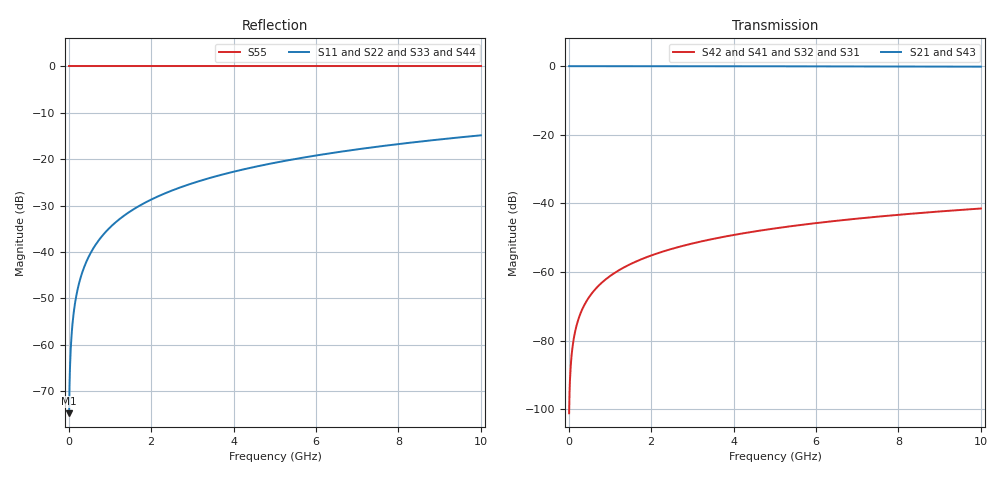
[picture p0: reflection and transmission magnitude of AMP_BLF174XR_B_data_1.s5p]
! Created Fri Oct  2 15:49:02 2009
# ghz S ma R 50
! 5 Port Network Data from SP1.SP block
! freq  magS11  angS11  magS12  angS12  magS13  angS13  magS14  angS14
!  magS15  angS15
!  magS21  angS21  magS22  angS22  magS23  angS23
!  magS24  angS24  magS25  angS25
!  magS31  angS31  magS32  angS32
!  magS33  angS33  magS34  angS34  magS35  angS35
!  magS41  angS41
!  magS42  angS42  magS43  angS43  magS44  angS44  magS45  angS45
!  magS51  angS51  magS52  angS52  magS53  angS53  magS54  angS54
!  magS55  angS55
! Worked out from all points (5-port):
!   1000 points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, 10 MHz to 10 GHz, reference 50 ohm
!   strongest paths, dB at 10 MHz, 2.51 GHz, 5.01 GHz, 7.51 GHz, 10 GHz:
!     S21: 0.0, 0.0, 0.0, -0.1, -0.1
!     S43: 0.0, 0.0, 0.0, -0.1, -0.1
!     S42: -101.2, -53.2, -47.3, -43.9, -41.5
!     S41: -101.2, -53.2, -47.3, -43.9, -41.5
!     S32: -101.2, -53.2, -47.3, -43.9, -41.5
!     S31: -101.2, -53.2, -47.3, -43.9, -41.5
!   lowest |S11| = -74.7 dB at 10 MHz (marker M1), VSWR 1.00, Z = 50 + j0.0183 ohm
!   |S11| at or under -10 dB: start of sweep to end of sweep
